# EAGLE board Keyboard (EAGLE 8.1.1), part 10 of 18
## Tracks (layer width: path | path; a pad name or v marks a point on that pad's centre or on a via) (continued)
S$9915 (continued)
  Bottom 0: 313.55,29.82 313.69,30.11
S$9916
  Bottom 0: 313.69,30.11 313.74,30.43
S$9917
  Bottom 0: 313.74,30.43 313.69,30.74
S$9918
  Bottom 0: 313.69,30.74 313.55,31.03
S$9919
  Bottom 0: 313.55,31.03 313.33,31.27
S$9920
  Bottom 0: 313.33,31.27 313.05,31.43
S$9921
  Bottom 0: 313.05,31.43 312.74,31.5
S$9922
  Bottom 0: 312.74,31.5 312.42,31.48
S$9923
  Bottom 0: 312.42,31.48 312.12,31.36
S$9924
  Bottom 0: 312.12,31.36 311.87,31.16
S$9925
  Bottom 0: 311.87,31.16 311.69,30.89
S$9926
  Bottom 0: 311.69,30.89 311.59,30.59
S$9927
  Bottom 0: 311.59,30.59 311.59,30.26
S$9928
  Bottom 0: 311.59,30.26 311.69,29.96
S$9929
  Bottom 0: 311.69,29.96 311.87,29.7
S$9930
  Bottom 0: 311.87,29.7 312.12,29.49
S$9931
  Bottom 0: 312.12,29.49 312.42,29.38
S$9932
  Bottom 0: 312.42,29.38 312.74,29.36
S$9933
  Bottom 0: 312.74,33.86 313.05,33.93
S$9934
  Bottom 0: 313.05,33.93 313.33,34.08
S$9935
  Bottom 0: 313.33,34.08 313.55,34.32
S$9936
  Bottom 0: 313.55,34.32 313.69,34.61
S$9937
  Bottom 0: 313.69,34.61 313.74,34.93
S$9938
  Bottom 0: 313.74,34.93 313.69,35.24
S$9939
  Bottom 0: 313.69,35.24 313.55,35.53
S$9940
  Bottom 0: 313.55,35.53 313.33,35.77
S$9941
  Bottom 0: 313.33,35.77 313.05,35.93
S$9942
  Bottom 0: 313.05,35.93 312.74,36
S$9943
  Bottom 0: 312.74,36 312.42,35.98
S$9944
  Bottom 0: 312.42,35.98 312.12,35.86
S$9945
  Bottom 0: 312.12,35.86 311.87,35.66
S$9946
  Bottom 0: 311.87,35.66 311.69,35.4
S$9947
  Bottom 0: 311.69,35.4 311.59,35.09
S$9948
  Bottom 0: 311.59,35.09 311.59,34.77
S$9949
  Bottom 0: 311.59,34.77 311.69,34.46
S$9950
  Bottom 0: 311.69,34.46 311.87,34.2
S$9951
  Bottom 0: 311.87,34.2 312.12,33.99
S$9952
  Bottom 0: 312.12,33.99 312.42,33.88
S$9953
  Bottom 0: 312.42,33.88 312.74,33.86
S$9954
  Bottom 0: 306.57,33.94 306.83,34.08
S$9955
  Bottom 0: 306.83,34.08 307.05,34.32
S$9956
  Bottom 0: 307.05,34.32 307.14,34.52
S$9957
  Bottom 0: 307.14,34.52 306.57,34.52
S$9958
  Bottom 0: 306.57,34.52 306.57,33.94
S$9959
  Bottom 0: 305.75,33.94 305.75,34.52
S$9960
  Bottom 0: 305.75,34.52 305.17,34.52
S$9961
  Bottom 0: 305.17,34.52 305.19,34.46
S$9962
  Bottom 0: 305.19,34.46 305.37,34.2
S$9963
  Bottom 0: 305.37,34.2 305.62,33.99
S$9964
  Bottom 0: 305.62,33.99 305.75,33.94
S$9965
  Bottom 0: 306.57,35.34 307.14,35.34
S$9966
  Bottom 0: 307.14,35.34 307.05,35.53
S$9967
  Bottom 0: 307.05,35.53 306.83,35.77
S$9968
  Bottom 0: 306.83,35.77 306.57,35.92
S$9969
  Bottom 0: 306.57,35.92 306.57,35.34
S$9970
  Bottom 0: 305.17,35.34 305.75,35.34
S$9971
  Bottom 0: 305.75,35.34 305.75,35.91
S$9972
  Bottom 0: 305.75,35.91 305.62,35.86
S$9973
  Bottom 0: 305.62,35.86 305.37,35.66
S$9974
  Bottom 0: 305.37,35.66 305.19,35.4
S$9975
  Bottom 0: 305.19,35.4 305.17,35.34
S$9976
  Bottom 0: 301.75,36.84 302.07,36.86
S$9977
  Bottom 0: 302.07,36.86 302.38,36.97
S$9978
  Bottom 0: 302.38,36.97 302.64,37.16
S$9979
  Bottom 0: 302.64,37.16 302.85,37.41
S$9980
  Bottom 0: 302.85,37.41 302.98,37.71
S$9981
  Bottom 0: 302.98,37.71 303.02,38.03
S$9982
  Bottom 0: 303.02,38.03 302.98,38.35
S$9983
  Bottom 0: 302.98,38.35 302.85,38.65
S$9984
  Bottom 0: 302.85,38.65 302.64,38.91
S$9985
  Bottom 0: 302.64,38.91 302.38,39.09
S$9986
  Bottom 0: 302.38,39.09 302.07,39.2
S$9987
  Bottom 0: 302.07,39.2 301.75,39.22
S$9988
  Bottom 0: 301.75,39.22 301.43,39.15
S$9989
  Bottom 0: 301.43,39.15 301.14,39.01
S$9990
  Bottom 0: 301.14,39.01 300.91,38.78
S$9991
  Bottom 0: 300.91,38.78 300.73,38.51
S$9992
  Bottom 0: 300.73,38.51 300.65,38.19
S$9993
  Bottom 0: 300.65,38.19 300.65,37.87
S$9994
  Bottom 0: 300.65,37.87 300.73,37.55
S$9995
  Bottom 0: 300.73,37.55 300.91,37.28
S$9996
  Bottom 0: 300.91,37.28 301.14,37.06
S$9997
  Bottom 0: 301.14,37.06 301.43,36.91
S$9998
  Bottom 0: 301.43,36.91 301.75,36.84
S$9999
  Bottom 0: 304.29,36.84 304.62,36.86
S$10000
  Bottom 0: 304.62,36.86 304.92,36.97
S$10001
  Bottom 0: 304.92,36.97 305.18,37.16
S$10002
  Bottom 0: 305.18,37.16 305.39,37.41
S$10003
  Bottom 0: 305.39,37.41 305.52,37.71
S$10004
  Bottom 0: 305.52,37.71 305.56,38.03
S$10005
  Bottom 0: 305.56,38.03 305.52,38.35
S$10006
  Bottom 0: 305.52,38.35 305.39,38.65
S$10007
  Bottom 0: 305.39,38.65 305.18,38.91
S$10008
  Bottom 0: 305.18,38.91 304.92,39.09
S$10009
  Bottom 0: 304.92,39.09 304.62,39.2
S$10010
  Bottom 0: 304.62,39.2 304.29,39.22
S$10011
  Bottom 0: 304.29,39.22 303.97,39.15
S$10012
  Bottom 0: 303.97,39.15 303.68,39.01
S$10013
  Bottom 0: 303.68,39.01 303.45,38.78
S$10014
  Bottom 0: 303.45,38.78 303.27,38.51
S$10015
  Bottom 0: 303.27,38.51 303.19,38.19
S$10016
  Bottom 0: 303.19,38.19 303.19,37.87
S$10017
  Bottom 0: 303.19,37.87 303.27,37.55
S$10018
  Bottom 0: 303.27,37.55 303.45,37.28
S$10019
  Bottom 0: 303.45,37.28 303.68,37.06
S$10020
  Bottom 0: 303.68,37.06 303.97,36.91
S$10021
  Bottom 0: 303.97,36.91 304.29,36.84
S$10022
  Bottom 0: 309.37,36.84 309.69,36.86
S$10023
  Bottom 0: 309.69,36.86 310,36.97
S$10024
  Bottom 0: 310,36.97 310.26,37.16
S$10025
  Bottom 0: 310.26,37.16 310.47,37.41
S$10026
  Bottom 0: 310.47,37.41 310.6,37.71
S$10027
  Bottom 0: 310.6,37.71 310.64,38.03
S$10028
  Bottom 0: 310.64,38.03 310.6,38.35
S$10029
  Bottom 0: 310.6,38.35 310.47,38.65
S$10030
  Bottom 0: 310.47,38.65 310.26,38.91
S$10031
  Bottom 0: 310.26,38.91 310,39.09
S$10032
  Bottom 0: 310,39.09 309.69,39.2
S$10033
  Bottom 0: 309.69,39.2 309.37,39.22
S$10034
  Bottom 0: 309.37,39.22 309.05,39.15
S$10035
  Bottom 0: 309.05,39.15 308.76,39.01
S$10036
  Bottom 0: 308.76,39.01 308.53,38.78
S$10037
  Bottom 0: 308.53,38.78 308.35,38.51
S$10038
  Bottom 0: 308.35,38.51 308.27,38.19
S$10039
  Bottom 0: 308.27,38.19 308.27,37.87
S$10040
  Bottom 0: 308.27,37.87 308.35,37.55
S$10041
  Bottom 0: 308.35,37.55 308.53,37.28
S$10042
  Bottom 0: 308.53,37.28 308.76,37.06
S$10043
  Bottom 0: 308.76,37.06 309.05,36.91
S$10044
  Bottom 0: 309.05,36.91 309.37,36.84
S$10045
  Bottom 0: 289.6,36.94 289.68,36.97
S$10046
  Bottom 0: 289.68,36.97 289.94,37.16
S$10047
  Bottom 0: 289.94,37.16 290.15,37.41
S$10048
  Bottom 0: 290.15,37.41 290.21,37.56
S$10049
  Bottom 0: 290.21,37.56 289.6,37.56
S$10050
  Bottom 0: 289.6,37.56 289.6,36.94
S$10051
  Bottom 0: 288.66,36.94 288.66,37.56
S$10052
  Bottom 0: 288.66,37.56 288.03,37.56
S$10053
  Bottom 0: 288.03,37.56 288.03,37.55
S$10054
  Bottom 0: 288.03,37.55 288.21,37.28
S$10055
  Bottom 0: 288.21,37.28 288.44,37.06
S$10056
  Bottom 0: 288.44,37.06 288.66,36.94
S$10057
  Bottom 0: 289.6,38.5 290.21,38.5
S$10058
  Bottom 0: 290.21,38.5 290.15,38.65
S$10059
  Bottom 0: 290.15,38.65 289.94,38.91
S$10060
  Bottom 0: 289.94,38.91 289.68,39.09
S$10061
  Bottom 0: 289.68,39.09 289.6,39.12
S$10062
  Bottom 0: 289.6,39.12 289.6,38.5
S$10063
  Bottom 0: 288.03,38.5 288.66,38.5
S$10064
  Bottom 0: 288.66,38.5 288.66,39.12
S$10065
  Bottom 0: 288.66,39.12 288.44,39.01
S$10066
  Bottom 0: 288.44,39.01 288.21,38.78
S$10067
  Bottom 0: 288.21,38.78 288.03,38.51
S$10068
  Bottom 0: 288.03,38.51 288.03,38.5
S$10069
  Bottom 0: 292.8,40.93 293.05,40.99
S$10070
  Bottom 0: 293.05,40.99 293.25,41.15
S$10071
  Bottom 0: 293.25,41.15 293.38,41.36
S$10072
  Bottom 0: 293.38,41.36 293.43,41.6
S$10073
  Bottom 0: 293.43,41.6 293.38,41.86
S$10074
  Bottom 0: 293.38,41.86 293.25,42.07
S$10075
  Bottom 0: 293.25,42.07 293.18,42.12
S$10076
  Bottom 0: 293.18,42.12 293.18,43.99
S$10077
  Bottom 0: 293.18,43.99 301.37,52.18
S$10078
  Bottom 0: 301.37,52.18 301.43,52.15
S$10079
  Bottom 0: 301.43,52.15 301.75,52.08
S$10080
  Bottom 0: 301.75,52.08 302.07,52.1
S$10081
  Bottom 0: 302.07,52.1 302.38,52.21
S$10082
  Bottom 0: 302.38,52.21 302.64,52.4
S$10083
  Bottom 0: 302.64,52.4 302.85,52.65
S$10084
  Bottom 0: 302.85,52.65 302.98,52.95
S$10085
  Bottom 0: 302.98,52.95 303.02,53.27
S$10086
  Bottom 0: 303.02,53.27 302.98,53.59
S$10087
  Bottom 0: 302.98,53.59 302.85,53.89
S$10088
  Bottom 0: 302.85,53.89 302.64,54.15
S$10089
  Bottom 0: 302.64,54.15 302.38,54.33
S$10090
  Bottom 0: 302.38,54.33 302.07,54.44
S$10091
  Bottom 0: 302.07,54.44 301.75,54.46
S$10092
  Bottom 0: 301.75,54.46 301.43,54.39
S$10093
  Bottom 0: 301.43,54.39 301.14,54.24
S$10094
  Bottom 0: 301.14,54.24 300.91,54.02
S$10095
  Bottom 0: 300.91,54.02 300.73,53.75
S$10096
  Bottom 0: 300.73,53.75 300.65,53.43
S$10097
  Bottom 0: 300.65,53.43 300.65,53.11
S$10098
  Bottom 0: 300.65,53.11 300.73,52.8
S$10099
  Bottom 0: 300.73,52.8 292.42,44.5
S$10100
  Bottom 0: 292.42,44.5 292.34,44.39
S$10101
  Bottom 0: 292.34,44.39 292.31,44.32
S$10102
  Bottom 0: 292.31,44.32 292.3,44.25
S$10103
  Bottom 0: 292.3,44.25 292.3,44.18
S$10104
  Bottom 0: 292.3,44.18 292.3,42.11
S$10105
  Bottom 0: 292.3,42.11 292.16,41.97
S$10106
  Bottom 0: 292.16,41.97 292.06,41.73
S$10107
  Bottom 0: 292.06,41.73 292.06,41.48
S$10108
  Bottom 0: 292.06,41.48 292.16,41.25
S$10109
  Bottom 0: 292.16,41.25 292.33,41.06
S$10110
  Bottom 0: 292.33,41.06 292.56,40.95
S$10111
  Bottom 0: 292.56,40.95 292.8,40.93
S$10112
  Bottom 0: 311.91,52.08 312.24,52.1
S$10113
  Bottom 0: 312.24,52.1 312.54,52.21
S$10114
  Bottom 0: 312.54,52.21 312.8,52.4
S$10115
  Bottom 0: 312.8,52.4 313.01,52.65
S$10116
  Bottom 0: 313.01,52.65 313.14,52.95
S$10117
  Bottom 0: 313.14,52.95 313.19,53.27
S$10118
  Bottom 0: 313.19,53.27 313.14,53.59
S$10119
  Bottom 0: 313.14,53.59 313.01,53.89
S$10120
  Bottom 0: 313.01,53.89 312.8,54.15
S$10121
  Bottom 0: 312.8,54.15 312.54,54.33
S$10122
  Bottom 0: 312.54,54.33 312.24,54.44
S$10123
  Bottom 0: 312.24,54.44 311.91,54.46
S$10124
  Bottom 0: 311.91,54.46 311.59,54.39
S$10125
  Bottom 0: 311.59,54.39 311.3,54.24
S$10126
  Bottom 0: 311.3,54.24 311.07,54.02
S$10127
  Bottom 0: 311.07,54.02 310.89,53.75
S$10128
  Bottom 0: 310.89,53.75 310.81,53.43
S$10129
  Bottom 0: 310.81,53.43 310.81,53.11
S$10130
  Bottom 0: 310.81,53.11 310.89,52.79
S$10131
  Bottom 0: 310.89,52.79 311.07,52.52
S$10132
  Bottom 0: 311.07,52.52 311.3,52.3
S$10133
  Bottom 0: 311.3,52.3 311.59,52.15
S$10134
  Bottom 0: 311.59,52.15 311.91,52.08
S$10135
  Bottom 0: 309.37,52.08 309.69,52.1
S$10136
  Bottom 0: 309.69,52.1 310,52.21
S$10137
  Bottom 0: 310,52.21 310.26,52.4
S$10138
  Bottom 0: 310.26,52.4 310.47,52.65
S$10139
  Bottom 0: 310.47,52.65 310.6,52.95
S$10140
  Bottom 0: 310.6,52.95 310.64,53.27
S$10141
  Bottom 0: 310.64,53.27 310.6,53.59
S$10142
  Bottom 0: 310.6,53.59 310.47,53.89
S$10143
  Bottom 0: 310.47,53.89 310.26,54.15
S$10144
  Bottom 0: 310.26,54.15 310,54.33
S$10145
  Bottom 0: 310,54.33 309.69,54.44
S$10146
  Bottom 0: 309.69,54.44 309.37,54.46
S$10147
  Bottom 0: 309.37,54.46 309.05,54.39
S$10148
  Bottom 0: 309.05,54.39 308.76,54.24
S$10149
  Bottom 0: 308.76,54.24 308.53,54.02
S$10150
  Bottom 0: 308.53,54.02 308.35,53.75
S$10151
  Bottom 0: 308.35,53.75 308.27,53.43
S$10152
  Bottom 0: 308.27,53.43 308.27,53.11
S$10153
  Bottom 0: 308.27,53.11 308.35,52.79
S$10154
  Bottom 0: 308.35,52.79 308.53,52.52
S$10155
  Bottom 0: 308.53,52.52 308.76,52.3
S$10156
  Bottom 0: 308.76,52.3 309.05,52.15
S$10157
  Bottom 0: 309.05,52.15 309.37,52.08
S$10158
  Bottom 0: 299.21,52.08 299.54,52.1
S$10159
  Bottom 0: 299.54,52.1 299.84,52.21
S$10160
  Bottom 0: 299.84,52.21 300.1,52.4
S$10161
  Bottom 0: 300.1,52.4 300.31,52.65
S$10162
  Bottom 0: 300.31,52.65 300.44,52.95
S$10163
  Bottom 0: 300.44,52.95 300.49,53.27
S$10164
  Bottom 0: 300.49,53.27 300.44,53.59
S$10165
  Bottom 0: 300.44,53.59 300.38,53.73
S$10166
  Bottom 0: 300.38,53.73 301.41,54.77
S$10167
  Bottom 0: 301.41,54.77 301.45,54.83
S$10168
  Bottom 0: 301.45,54.83 301.5,54.88
S$10169
  Bottom 0: 301.5,54.88 301.52,54.95
S$10170
  Bottom 0: 301.52,54.95 301.54,55.01
S$10171
  Bottom 0: 301.54,55.01 301.54,55.09
S$10172
  Bottom 0: 301.54,55.09 301.54,60.8
S$10173
  Bottom 0: 301.54,60.8 301.6,60.78
S$10174
  Bottom 0: 301.6,60.78 301.95,60.76
S$10175
  Bottom 0: 301.95,60.76 302.29,60.82
S$10176
  Bottom 0: 302.29,60.82 302.61,60.97
S$10177
  Bottom 0: 302.61,60.97 302.88,61.2
S$10178
  Bottom 0: 302.88,61.2 303.09,61.48
S$10179
  Bottom 0: 303.09,61.48 303.21,61.81
S$10180
  Bottom 0: 303.21,61.81 303.26,62.15
S$10181
  Bottom 0: 303.26,62.15 303.21,62.49
S$10182
  Bottom 0: 303.21,62.49 303.09,62.82
S$10183
  Bottom 0: 303.09,62.82 302.88,63.11
S$10184
  Bottom 0: 302.88,63.11 302.61,63.33
S$10185
  Bottom 0: 302.61,63.33 302.29,63.48
S$10186
  Bottom 0: 302.29,63.48 301.95,63.54
S$10187
  Bottom 0: 301.95,63.54 301.6,63.52
S$10188
  Bottom 0: 301.6,63.52 301.49,63.49
S$10189
  Bottom 0: 301.49,63.49 301.19,63.54
S$10190
  Bottom 0: 301.19,63.54 300.83,63.52
S$10191
  Bottom 0: 300.83,63.52 300.5,63.41
S$10192
  Bottom 0: 300.5,63.41 300.21,63.23
S$10193
  Bottom 0: 300.21,63.23 299.97,62.97
S$10194
  Bottom 0: 299.97,62.97 299.8,62.66
S$10195
  Bottom 0: 299.8,62.66 299.71,62.32
S$10196
  Bottom 0: 299.71,62.32 299.71,61.98
S$10197
  Bottom 0: 299.71,61.98 299.8,61.64
S$10198
  Bottom 0: 299.8,61.64 299.97,61.33
S$10199
  Bottom 0: 299.97,61.33 300.21,61.07
S$10200
  Bottom 0: 300.21,61.07 300.5,60.89
S$10201
  Bottom 0: 300.5,60.89 300.66,60.84
S$10202
  Bottom 0: 300.66,60.84 300.66,55.27
S$10203
  Bottom 0: 300.66,55.27 299.75,54.36
S$10204
  Bottom 0: 299.75,54.36 299.54,54.44
S$10205
  Bottom 0: 299.54,54.44 299.21,54.46
S$10206
  Bottom 0: 299.21,54.46 298.89,54.39
S$10207
  Bottom 0: 298.89,54.39 298.6,54.24
S$10208
  Bottom 0: 298.6,54.24 298.37,54.02
S$10209
  Bottom 0: 298.37,54.02 298.19,53.75
S$10210
  Bottom 0: 298.19,53.75 298.11,53.43
S$10211
  Bottom 0: 298.11,53.43 298.11,53.11
S$10212
  Bottom 0: 298.11,53.11 298.19,52.79
S$10213
  Bottom 0: 298.19,52.79 298.37,52.52
S$10214
  Bottom 0: 298.37,52.52 298.6,52.3
S$10215
  Bottom 0: 298.6,52.3 298.89,52.15
S$10216
  Bottom 0: 298.89,52.15 299.21,52.08
S$10217
  Bottom 0: 296.67,52.08 297,52.1
S$10218
  Bottom 0: 297,52.1 297.3,52.21
S$10219
  Bottom 0: 297.3,52.21 297.56,52.4
S$10220
  Bottom 0: 297.56,52.4 297.77,52.65
S$10221
  Bottom 0: 297.77,52.65 297.9,52.95
S$10222
  Bottom 0: 297.9,52.95 297.94,53.27
S$10223
  Bottom 0: 297.94,53.27 297.9,53.59
S$10224
  Bottom 0: 297.9,53.59 297.77,53.89
S$10225
  Bottom 0: 297.77,53.89 297.56,54.15
S$10226
  Bottom 0: 297.56,54.15 297.3,54.33
S$10227
  Bottom 0: 297.3,54.33 297,54.44
S$10228
  Bottom 0: 297,54.44 296.67,54.46
S$10229
  Bottom 0: 296.67,54.46 296.35,54.39
S$10230
  Bottom 0: 296.35,54.39 296.06,54.24
S$10231
  Bottom 0: 296.06,54.24 295.83,54.02
S$10232
  Bottom 0: 295.83,54.02 295.65,53.75
S$10233
  Bottom 0: 295.65,53.75 295.57,53.43
S$10234
  Bottom 0: 295.57,53.43 295.57,53.11
S$10235
  Bottom 0: 295.57,53.11 295.65,52.79
S$10236
  Bottom 0: 295.65,52.79 295.83,52.52
S$10237
  Bottom 0: 295.83,52.52 296.06,52.3
S$10238
  Bottom 0: 296.06,52.3 296.35,52.15
S$10239
  Bottom 0: 296.35,52.15 296.67,52.08
S$10240
  Bottom 0: 289.05,52.08 289.38,52.1
S$10241
  Bottom 0: 289.38,52.1 289.68,52.21
S$10242
  Bottom 0: 289.68,52.21 289.94,52.4
S$10243
  Bottom 0: 289.94,52.4 290.15,52.65
S$10244
  Bottom 0: 290.15,52.65 290.28,52.95
S$10245
  Bottom 0: 290.28,52.95 290.32,53.27
S$10246
  Bottom 0: 290.32,53.27 290.28,53.59
S$10247
  Bottom 0: 290.28,53.59 290.15,53.89
S$10248
  Bottom 0: 290.15,53.89 289.94,54.15
S$10249
  Bottom 0: 289.94,54.15 289.68,54.33
S$10250
  Bottom 0: 289.68,54.33 289.38,54.44
S$10251
  Bottom 0: 289.38,54.44 289.05,54.46
S$10252
  Bottom 0: 289.05,54.46 288.73,54.39
S$10253
  Bottom 0: 288.73,54.39 288.44,54.24
S$10254
  Bottom 0: 288.44,54.24 288.21,54.02
S$10255
  Bottom 0: 288.21,54.02 288.03,53.75
S$10256
  Bottom 0: 288.03,53.75 287.95,53.43
S$10257
  Bottom 0: 287.95,53.43 287.95,53.11
S$10258
  Bottom 0: 287.95,53.11 288.03,52.79
S$10259
  Bottom 0: 288.03,52.79 288.21,52.52
S$10260
  Bottom 0: 288.21,52.52 288.44,52.3
S$10261
  Bottom 0: 288.44,52.3 288.73,52.15
S$10262
  Bottom 0: 288.73,52.15 289.05,52.08
S$10263
  Bottom 0: 286.51,52.08 286.83,52.1
S$10264
  Bottom 0: 286.83,52.1 287.14,52.21
S$10265
  Bottom 0: 287.14,52.21 287.4,52.4
S$10266
  Bottom 0: 287.4,52.4 287.61,52.65
S$10267
  Bottom 0: 287.61,52.65 287.74,52.95
S$10268
  Bottom 0: 287.74,52.95 287.79,53.27
S$10269
  Bottom 0: 287.79,53.27 287.74,53.59
S$10270
  Bottom 0: 287.74,53.59 287.61,53.89
S$10271
  Bottom 0: 287.61,53.89 287.4,54.15
S$10272
  Bottom 0: 287.4,54.15 287.14,54.33
S$10273
  Bottom 0: 287.14,54.33 286.83,54.44
S$10274
  Bottom 0: 286.83,54.44 286.51,54.46
S$10275
  Bottom 0: 286.51,54.46 286.19,54.39
S$10276
  Bottom 0: 286.19,54.39 285.9,54.24
S$10277
  Bottom 0: 285.9,54.24 285.67,54.02
S$10278
  Bottom 0: 285.67,54.02 285.49,53.75
S$10279
  Bottom 0: 285.49,53.75 285.41,53.43
S$10280
  Bottom 0: 285.41,53.43 285.41,53.11
S$10281
  Bottom 0: 285.41,53.11 285.49,52.79
S$10282
  Bottom 0: 285.49,52.79 285.67,52.52
S$10283
  Bottom 0: 285.67,52.52 285.9,52.3
S$10284
  Bottom 0: 285.9,52.3 286.19,52.15
S$10285
  Bottom 0: 286.19,52.15 286.51,52.08
S$10286
  Bottom 0: 294.68,52.18 294.76,52.21
S$10287
  Bottom 0: 294.76,52.21 295.02,52.4
S$10288
  Bottom 0: 295.02,52.4 295.23,52.65
S$10289
  Bottom 0: 295.23,52.65 295.3,52.8
S$10290
  Bottom 0: 295.3,52.8 294.68,52.8
S$10291
  Bottom 0: 294.68,52.8 294.68,52.18
S$10292
  Bottom 0: 292.14,52.18 292.22,52.21
S$10293
  Bottom 0: 292.22,52.21 292.48,52.4
S$10294
  Bottom 0: 292.48,52.4 292.69,52.65
S$10295
  Bottom 0: 292.69,52.65 292.75,52.8
S$10296
  Bottom 0: 292.75,52.8 292.14,52.8
S$10297
  Bottom 0: 292.14,52.8 292.14,52.18
S$10298
  Bottom 0: 293.74,52.18 293.74,52.8
S$10299
  Bottom 0: 293.74,52.8 293.11,52.8
S$10300
  Bottom 0: 293.11,52.8 293.11,52.79
S$10301
  Bottom 0: 293.11,52.79 293.29,52.52
S$10302
  Bottom 0: 293.29,52.52 293.52,52.3
S$10303
  Bottom 0: 293.52,52.3 293.74,52.18
S$10304
  Bottom 0: 291.2,52.18 291.2,52.8
S$10305
  Bottom 0: 291.2,52.8 290.57,52.8
S$10306
  Bottom 0: 290.57,52.8 290.57,52.79
S$10307
  Bottom 0: 290.57,52.79 290.75,52.52
S$10308
  Bottom 0: 290.75,52.52 290.98,52.3
S$10309
  Bottom 0: 290.98,52.3 291.2,52.18
S$10310
  Bottom 0: 294.68,53.74 295.3,53.74
S$10311
  Bottom 0: 295.3,53.74 295.23,53.89
S$10312
  Bottom 0: 295.23,53.89 295.02,54.15
S$10313
  Bottom 0: 295.02,54.15 294.76,54.33
S$10314
  Bottom 0: 294.76,54.33 294.68,54.36
S$10315
  Bottom 0: 294.68,54.36 294.68,53.74
S$10316
  Bottom 0: 293.11,53.74 293.74,53.74
S$10317
  Bottom 0: 293.74,53.74 293.74,54.36
S$10318
  Bottom 0: 293.74,54.36 293.52,54.24
S$10319
  Bottom 0: 293.52,54.24 293.29,54.02
S$10320
  Bottom 0: 293.29,54.02 293.11,53.75
S$10321
  Bottom 0: 293.11,53.75 293.11,53.74
S$10322
  Bottom 0: 292.14,53.74 292.75,53.74
S$10323
  Bottom 0: 292.75,53.74 292.69,53.89
S$10324
  Bottom 0: 292.69,53.89 292.48,54.15
S$10325
  Bottom 0: 292.48,54.15 292.22,54.33
S$10326
  Bottom 0: 292.22,54.33 292.14,54.36
S$10327
  Bottom 0: 292.14,54.36 292.14,53.74
S$10328
  Bottom 0: 290.57,53.74 291.2,53.74
S$10329
  Bottom 0: 291.2,53.74 291.2,54.36
S$10330
  Bottom 0: 291.2,54.36 290.98,54.24
S$10331
  Bottom 0: 290.98,54.24 290.75,54.02
S$10332
  Bottom 0: 290.75,54.02 290.57,53.75
S$10333
  Bottom 0: 290.57,53.75 290.57,53.74
S$10334
  Bottom 0: 294.84,58.22 295.14,58.27
S$10335
  Bottom 0: 295.14,58.27 295.25,58.24
S$10336
  Bottom 0: 295.25,58.24 295.6,58.22
S$10337
  Bottom 0: 295.6,58.22 295.94,58.28
S$10338
  Bottom 0: 295.94,58.28 296.25,58.43
S$10339
  Bottom 0: 296.25,58.43 296.53,58.66
S$10340
  Bottom 0: 296.53,58.66 296.74,58.94
S$10341
  Bottom 0: 296.74,58.94 296.86,59.27
S$10342
  Bottom 0: 296.86,59.27 296.91,59.61
S$10343
  Bottom 0: 296.91,59.61 296.86,59.95
S$10344
  Bottom 0: 296.86,59.95 296.74,60.28
S$10345
  Bottom 0: 296.74,60.28 296.53,60.57
S$10346
  Bottom 0: 296.53,60.57 296.25,60.79
S$10347
  Bottom 0: 296.25,60.79 295.94,60.94
S$10348
  Bottom 0: 295.94,60.94 295.6,61
S$10349
  Bottom 0: 295.6,61 295.25,60.98
S$10350
  Bottom 0: 295.25,60.98 295.14,60.95
S$10351
  Bottom 0: 295.14,60.95 294.84,61
S$10352
  Bottom 0: 294.84,61 294.49,60.98
S$10353
  Bottom 0: 294.49,60.98 294.15,60.87
S$10354
  Bottom 0: 294.15,60.87 293.86,60.69
S$10355
  Bottom 0: 293.86,60.69 293.62,60.43
S$10356
  Bottom 0: 293.62,60.43 293.45,60.12
S$10357
  Bottom 0: 293.45,60.12 293.43,60.05
S$10358
  Bottom 0: 293.43,60.05 290.28,60.05
S$10359
  Bottom 0: 290.28,60.05 289.52,60.8
S$10360
  Bottom 0: 289.52,60.8 289.54,60.83
S$10361
  Bottom 0: 289.54,60.83 289.58,61.13
S$10362
  Bottom 0: 289.58,61.13 289.54,61.43
S$10363
  Bottom 0: 289.54,61.43 289.41,61.7
S$10364
  Bottom 0: 289.41,61.7 289.2,61.92
S$10365
  Bottom 0: 289.2,61.92 288.94,62.08
S$10366
  Bottom 0: 288.94,62.08 288.65,62.14
S$10367
  Bottom 0: 288.65,62.14 288.34,62.12
S$10368
  Bottom 0: 288.34,62.12 288.06,62.01
S$10369
  Bottom 0: 288.06,62.01 287.82,61.82
S$10370
  Bottom 0: 287.82,61.82 287.66,61.57
S$10371
  Bottom 0: 287.66,61.57 287.57,61.28
S$10372
  Bottom 0: 287.57,61.28 287.57,60.98
S$10373
  Bottom 0: 287.57,60.98 287.66,60.69
S$10374
  Bottom 0: 287.66,60.69 287.82,60.44
S$10375
  Bottom 0: 287.82,60.44 288.06,60.25
S$10376
  Bottom 0: 288.06,60.25 288.34,60.14
S$10377
  Bottom 0: 288.34,60.14 288.65,60.12
S$10378
  Bottom 0: 288.65,60.12 288.9,60.17
S$10379
  Bottom 0: 288.9,60.17 289.77,59.3
S$10380
  Bottom 0: 289.77,59.3 289.83,59.26
S$10381
  Bottom 0: 289.83,59.26 289.89,59.22
S$10382
  Bottom 0: 289.89,59.22 289.95,59.19
S$10383
  Bottom 0: 289.95,59.19 290.02,59.17
S$10384
  Bottom 0: 290.02,59.17 290.09,59.17
S$10385
  Bottom 0: 290.09,59.17 293.43,59.17
S$10386
  Bottom 0: 293.43,59.17 293.45,59.1
S$10387
  Bottom 0: 293.45,59.1 293.62,58.79
S$10388
  Bottom 0: 293.62,58.79 293.86,58.53
S$10389
  Bottom 0: 293.86,58.53 294.15,58.35
S$10390
  Bottom 0: 294.15,58.35 294.49,58.24
S$10391
  Bottom 0: 294.49,58.24 294.84,58.22
S$10392
  Bottom 0: 297.29,62.41 297.67,62.45
S$10393
  Bottom 0: 297.67,62.45 298.05,62.41
S$10394
  Bottom 0: 298.05,62.41 298.5,62.45
S$10395
  Bottom 0: 298.5,62.45 298.92,62.58
S$10396
  Bottom 0: 298.92,62.58 299.32,62.79
S$10397
  Bottom 0: 299.32,62.79 299.67,63.08
S$10398
  Bottom 0: 299.67,63.08 299.95,63.42
S$10399
  Bottom 0: 299.95,63.42 300.16,63.82
S$10400
  Bottom 0: 300.16,63.82 300.29,64.24
S$10401
  Bottom 0: 300.29,64.24 300.34,64.69
S$10402
  Bottom 0: 300.34,64.69 300.29,65.14
S$10403
  Bottom 0: 300.29,65.14 300.16,65.56
S$10404
  Bottom 0: 300.16,65.56 299.95,65.96
S$10405
  Bottom 0: 299.95,65.96 299.67,66.3
S$10406
  Bottom 0: 299.67,66.3 299.32,66.59
S$10407
  Bottom 0: 299.32,66.59 298.92,66.81
S$10408
  Bottom 0: 298.92,66.81 298.5,66.93
S$10409
  Bottom 0: 298.5,66.93 298.05,66.98
S$10410
  Bottom 0: 298.05,66.98 297.67,66.94
S$10411
  Bottom 0: 297.67,66.94 297.29,66.98
S$10412
  Bottom 0: 297.29,66.98 296.84,66.93
S$10413
  Bottom 0: 296.84,66.93 296.42,66.81
S$10414
  Bottom 0: 296.42,66.81 296.02,66.59
S$10415
  Bottom 0: 296.02,66.59 295.67,66.3
S$10416
  Bottom 0: 295.67,66.3 295.39,65.96
S$10417
  Bottom 0: 295.39,65.96 295.17,65.56
S$10418
  Bottom 0: 295.17,65.56 295.05,65.14
S$10419
  Bottom 0: 295.05,65.14 295,64.69
S$10420
  Bottom 0: 295,64.69 295.05,64.24
S$10421
  Bottom 0: 295.05,64.24 295.17,63.82
S$10422
  Bottom 0: 295.17,63.82 295.39,63.42
S$10423
  Bottom 0: 295.39,63.42 295.67,63.08
S$10424
  Bottom 0: 295.67,63.08 296.02,62.79
S$10425
  Bottom 0: 296.02,62.79 296.42,62.58
S$10426
  Bottom 0: 296.42,62.58 296.84,62.45
S$10427
  Bottom 0: 296.84,62.45 297.29,62.41
S$10428
  Bottom 0: 288.65,67.74 288.94,67.81
S$10429
  Bottom 0: 288.94,67.81 289.2,67.95
S$10430
  Bottom 0: 289.2,67.95 289.41,68.18
S$10431
  Bottom 0: 289.41,68.18 289.54,68.45
S$10432
  Bottom 0: 289.54,68.45 289.58,68.75
S$10433
  Bottom 0: 289.58,68.75 289.54,69.05
S$10434
  Bottom 0: 289.54,69.05 289.41,69.32
S$10435
  Bottom 0: 289.41,69.32 289.2,69.54
S$10436
  Bottom 0: 289.2,69.54 288.94,69.69
S$10437
  Bottom 0: 288.94,69.69 288.65,69.76
S$10438
  Bottom 0: 288.65,69.76 288.34,69.74
S$10439
  Bottom 0: 288.34,69.74 288.06,69.63
S$10440
  Bottom 0: 288.06,69.63 287.82,69.44
S$10441
  Bottom 0: 287.82,69.44 287.66,69.19
S$10442
  Bottom 0: 287.66,69.19 287.57,68.9
S$10443
  Bottom 0: 287.57,68.9 287.57,68.59
S$10444
  Bottom 0: 287.57,68.59 287.66,68.31
S$10445
  Bottom 0: 287.66,68.31 287.82,68.06
S$10446
  Bottom 0: 287.82,68.06 288.06,67.87
S$10447
  Bottom 0: 288.06,67.87 288.34,67.76
S$10448
  Bottom 0: 288.34,67.76 288.65,67.74
S$10449
  Bottom 0: 284.32,73.98 284.86,73.98
S$10450
  Bottom 0: 284.86,73.98 284.94,73.99
S$10451
  Bottom 0: 284.94,73.99 285.01,74.03
S$10452
  Bottom 0: 285.01,74.03 285.06,74.08
S$10453
  Bottom 0: 285.06,74.08 285.1,74.16
S$10454
  Bottom 0: 285.1,74.16 285.11,74.23
S$10455
  Bottom 0: 285.11,74.23 285.11,74.53
S$10456
  Bottom 0: 285.11,74.53 284.32,74.53
S$10457
  Bottom 0: 284.32,74.53 284.32,73.98
S$10458
  Bottom 0: 282.7,73.98 283.24,73.98
S$10459
  Bottom 0: 283.24,73.98 283.24,74.53
S$10460
  Bottom 0: 283.24,74.53 282.44,74.53
S$10461
  Bottom 0: 282.44,74.53 282.44,74.23
S$10462
  Bottom 0: 282.44,74.23 282.46,74.16
S$10463
  Bottom 0: 282.46,74.16 282.5,74.08
S$10464
  Bottom 0: 282.5,74.08 282.55,74.03
S$10465
  Bottom 0: 282.55,74.03 282.62,73.99
S$10466
  Bottom 0: 282.62,73.99 282.7,73.98
S$10467
  Bottom 0: 284.32,75.13 285.11,75.13
S$10468
  Bottom 0: 285.11,75.13 285.11,75.43
S$10469
  Bottom 0: 285.11,75.43 285.1,75.51
S$10470
  Bottom 0: 285.1,75.51 285.06,75.58
S$10471
  Bottom 0: 285.06,75.58 285.01,75.63
S$10472
  Bottom 0: 285.01,75.63 284.94,75.67
S$10473
  Bottom 0: 284.94,75.67 284.86,75.68
S$10474
  Bottom 0: 284.86,75.68 284.32,75.68
S$10475
  Bottom 0: 284.32,75.68 284.32,75.13
S$10476
  Bottom 0: 282.44,75.13 283.24,75.13
S$10477
  Bottom 0: 283.24,75.13 283.24,75.68
S$10478
  Bottom 0: 283.24,75.68 282.7,75.68
S$10479
  Bottom 0: 282.7,75.68 282.62,75.67
S$10480
  Bottom 0: 282.62,75.67 282.55,75.63
S$10481
  Bottom 0: 282.55,75.63 282.5,75.58
S$10482
  Bottom 0: 282.5,75.58 282.46,75.51
S$10483
  Bottom 0: 282.46,75.51 282.44,75.43
S$10484
  Bottom 0: 282.44,75.43 282.44,75.13
S$10485
  Bottom 0: 306.59,78.25 307.11,78.25
S$10486
  Bottom 0: 307.11,78.25 307.61,78.34
S$10487
  Bottom 0: 307.61,78.34 308.11,78.5
S$10488
  Bottom 0: 308.11,78.5 308.56,78.75
S$10489
  Bottom 0: 308.56,78.75 308.97,79.07
S$10490
  Bottom 0: 308.97,79.07 309.32,79.45
S$10491
  Bottom 0: 309.32,79.45 309.61,79.88
S$10492
  Bottom 0: 309.61,79.88 309.82,80.36
S$10493
  Bottom 0: 309.82,80.36 309.94,80.86
S$10494
  Bottom 0: 309.94,80.86 309.98,81.37
S$10495
  Bottom 0: 309.98,81.37 309.94,81.89
S$10496
  Bottom 0: 309.94,81.89 309.82,82.39
S$10497
  Bottom 0: 309.82,82.39 309.61,82.87
S$10498
  Bottom 0: 309.61,82.87 309.32,83.3
S$10499
  Bottom 0: 309.32,83.3 308.97,83.68
S$10500
  Bottom 0: 308.97,83.68 308.56,84
S$10501
  Bottom 0: 308.56,84 308.11,84.24
S$10502
  Bottom 0: 308.11,84.24 307.61,84.41
S$10503
  Bottom 0: 307.61,84.41 307.11,84.5
S$10504
  Bottom 0: 307.11,84.5 306.59,84.5
S$10505
  Bottom 0: 306.59,84.5 306.08,84.41
S$10506
  Bottom 0: 306.08,84.41 305.59,84.24
S$10507
  Bottom 0: 305.59,84.24 305.14,84
S$10508
  Bottom 0: 305.14,84 304.73,83.68
S$10509
  Bottom 0: 304.73,83.68 304.38,83.3
S$10510
  Bottom 0: 304.38,83.3 304.09,82.87
S$10511
  Bottom 0: 304.09,82.87 303.88,82.39
S$10512
  Bottom 0: 303.88,82.39 303.76,81.89
S$10513
  Bottom 0: 303.76,81.89 303.71,81.37
S$10514
  Bottom 0: 303.71,81.37 303.76,80.86
S$10515
  Bottom 0: 303.76,80.86 303.88,80.36
S$10516
  Bottom 0: 303.88,80.36 304.09,79.88
S$10517
  Bottom 0: 304.09,79.88 304.38,79.45
S$10518
  Bottom 0: 304.38,79.45 304.73,79.07
S$10519
  Bottom 0: 304.73,79.07 305.14,78.75
S$10520
  Bottom 0: 305.14,78.75 305.59,78.5
S$10521
  Bottom 0: 305.59,78.5 306.08,78.34
S$10522
  Bottom 0: 306.08,78.34 306.59,78.25
S$10523
  Bottom 0: 289.84,79.65 290.14,79.72
S$10524
  Bottom 0: 290.14,79.72 290.4,79.87
S$10525
  Bottom 0: 290.4,79.87 290.6,80.09
S$10526
  Bottom 0: 290.6,80.09 290.74,80.36
S$10527
  Bottom 0: 290.74,80.36 290.78,80.66
S$10528
  Bottom 0: 290.78,80.66 290.74,80.96
S$10529
  Bottom 0: 290.74,80.96 290.6,81.24
S$10530
  Bottom 0: 290.6,81.24 290.4,81.45
S$10531
  Bottom 0: 290.4,81.45 290.14,81.61
S$10532
  Bottom 0: 290.14,81.61 289.84,81.67
S$10533
  Bottom 0: 289.84,81.67 289.54,81.65
S$10534
  Bottom 0: 289.54,81.65 289.26,81.54
S$10535
  Bottom 0: 289.26,81.54 289.02,81.35
S$10536
  Bottom 0: 289.02,81.35 288.85,81.11
S$10537
  Bottom 0: 288.85,81.11 288.76,80.81
S$10538
  Bottom 0: 288.76,80.81 288.76,80.51
S$10539
  Bottom 0: 288.76,80.51 288.85,80.22
S$10540
  Bottom 0: 288.85,80.22 289.02,79.97
S$10541
  Bottom 0: 289.02,79.97 289.26,79.78
S$10542
  Bottom 0: 289.26,79.78 289.54,79.67
S$10543
  Bottom 0: 289.54,79.67 289.84,79.65
S$10544
  Bottom 0: 287.52,82.63 287.52,83.12
S$10545
  Bottom 0: 287.52,83.12 287.03,83.12
S$10546
  Bottom 0: 287.03,83.12 287.07,83.02
S$10547
  Bottom 0: 287.07,83.02 287.24,82.79
S$10548
  Bottom 0: 287.24,82.79 287.48,82.64
S$10549
  Bottom 0: 287.48,82.64 287.52,82.63
S$10550
  Bottom 0: 288.12,82.63 288.29,82.7
S$10551
  Bottom 0: 288.29,82.7 288.5,82.9
S$10552
  Bottom 0: 288.5,82.9 288.62,83.12
S$10553
  Bottom 0: 288.62,83.12 288.12,83.12
S$10554
  Bottom 0: 288.12,83.12 288.12,82.63
S$10555
  Bottom 0: 288.12,83.72 288.62,83.72
S$10556
  Bottom 0: 288.62,83.72 288.5,83.94
S$10557
  Bottom 0: 288.5,83.94 288.29,84.14
S$10558
  Bottom 0: 288.29,84.14 288.12,84.21
S$10559
  Bottom 0: 288.12,84.21 288.12,83.72
S$10560
  Bottom 0: 289.3,87.25 289.3,87.95
S$10561
  Bottom 0: 289.3,87.95 288.6,87.95
S$10562
  Bottom 0: 288.6,87.95 288.75,87.7
S$10563
  Bottom 0: 288.75,87.7 288.98,87.44
S$10564
  Bottom 0: 288.98,87.44 289.28,87.26
S$10565
  Bottom 0: 289.28,87.26 289.3,87.25
S$10566
  Bottom 0: 290.45,87.26 290.63,87.34
S$10567
  Bottom 0: 290.63,87.34 290.9,87.57
S$10568
  Bottom 0: 290.9,87.57 291.1,87.85
S$10569
  Bottom 0: 291.1,87.85 291.15,87.95
S$10570
  Bottom 0: 291.15,87.95 290.45,87.95
S$10571
  Bottom 0: 290.45,87.95 290.45,87.26
S$10572
  Bottom 0: 59.95,12.5 59.98,12.64
S$10573
  Bottom 0: 59.98,12.64 59.93,12.96
S$10574
  Bottom 0: 59.93,12.96 59.79,13.26
S$10575
  Bottom 0: 59.79,13.26 59.58,13.5
S$10576
  Bottom 0: 59.58,13.5 59.31,13.68
S$10577
  Bottom 0: 59.31,13.68 59,13.77
S$10578
  Bottom 0: 59,13.77 58.67,13.77
S$10579
  Bottom 0: 58.67,13.77 58.54,13.73
S$10580
  Bottom 0: 58.54,13.73 56.56,15.71
S$10581
  Bottom 0: 56.56,15.71 56.56,27.38
S$10582
  Bottom 0: 56.56,27.38 56.56,27.48
S$10583
  Bottom 0: 56.56,27.48 56.54,27.56
S$10584
  Bottom 0: 56.54,27.56 56.5,27.64
S$10585
  Bottom 0: 56.5,27.64 56.46,27.72
S$10586
  Bottom 0: 56.46,27.72 56.39,27.79
S$10587
  Bottom 0: 56.39,27.79 52.79,31.39
S$10588
  Bottom 0: 52.79,31.39 52.83,31.69
S$10589
  Bottom 0: 52.83,31.69 52.78,32.01
S$10590
  Bottom 0: 52.78,32.01 52.65,32.31
S$10591
  Bottom 0: 52.65,32.31 52.43,32.55
S$10592
  Bottom 0: 52.43,32.55 52.16,32.73
S$10593
  Bottom 0: 52.16,32.73 51.85,32.82
S$10594
  Bottom 0: 51.85,32.82 51.52,32.82
S$10595
  Bottom 0: 51.52,32.82 51.21,32.73
S$10596
  Bottom 0: 51.21,32.73 50.94,32.55
S$10597
  Bottom 0: 50.94,32.55 50.73,32.31
S$10598
  Bottom 0: 50.73,32.31 50.59,32.01
S$10599
  Bottom 0: 50.59,32.01 50.54,31.69
S$10600
  Bottom 0: 50.54,31.69 50.59,31.37
S$10601
  Bottom 0: 50.59,31.37 50.73,31.07
S$10602
  Bottom 0: 50.73,31.07 50.94,30.82
S$10603
  Bottom 0: 50.94,30.82 51.21,30.64
S$10604
  Bottom 0: 51.21,30.64 51.52,30.55
S$10605
  Bottom 0: 51.52,30.55 51.85,30.55
S$10606
  Bottom 0: 51.85,30.55 51.98,30.59
S$10607
  Bottom 0: 51.98,30.59 55.42,27.15
S$10608
  Bottom 0: 55.42,27.15 55.42,24.77
S$10609
  Bottom 0: 55.42,24.77 55.24,25.02
S$10610
  Bottom 0: 55.24,25.02 54.97,25.25
S$10611
  Bottom 0: 54.97,25.25 54.67,25.39
S$10612
  Bottom 0: 54.67,25.39 54.67,26.2
S$10613
  Bottom 0: 54.67,26.2 54.66,26.28
S$10614
  Bottom 0: 54.66,26.28 54.65,26.34
S$10615
  Bottom 0: 54.65,26.34 54.62,26.4
S$10616
  Bottom 0: 54.62,26.4 54.58,26.46
S$10617
  Bottom 0: 54.58,26.46 54.54,26.52
S$10618
  Bottom 0: 54.54,26.52 50.8,30.25
S$10619
  Bottom 0: 50.8,30.25 50.75,30.3
S$10620
  Bottom 0: 50.75,30.3 50.69,30.34
S$10621
  Bottom 0: 50.69,30.34 50.63,30.36
S$10622
  Bottom 0: 50.63,30.36 50.56,30.38
S$10623
  Bottom 0: 50.56,30.38 50.49,30.38
S$10624
  Bottom 0: 50.49,30.38 46.93,30.38
S$10625
  Bottom 0: 46.93,30.38 38.11,39.2
S$10626
  Bottom 0: 38.11,39.2 38.44,39.19
S$10627
  Bottom 0: 38.44,39.19 38.78,39.25
S$10628
  Bottom 0: 38.78,39.25 39.1,39.4
S$10629
  Bottom 0: 39.1,39.4 39.37,39.62
S$10630
  Bottom 0: 39.37,39.62 39.57,39.91
S$10631
  Bottom 0: 39.57,39.91 39.7,40.23
S$10632
  Bottom 0: 39.7,40.23 39.75,40.58
S$10633
  Bottom 0: 39.75,40.58 39.7,40.92
S$10634
  Bottom 0: 39.7,40.92 39.57,41.25
S$10635
  Bottom 0: 39.57,41.25 39.37,41.53
S$10636
  Bottom 0: 39.37,41.53 39.1,41.76
S$10637
  Bottom 0: 39.1,41.76 38.78,41.91
S$10638
  Bottom 0: 38.78,41.91 38.44,41.97
S$10639
  Bottom 0: 38.44,41.97 38.09,41.95
S$10640
  Bottom 0: 38.09,41.95 37.76,41.84
S$10641
  Bottom 0: 37.76,41.84 37.46,41.65
S$10642
  Bottom 0: 37.46,41.65 37.28,41.46
S$10643
  Bottom 0: 37.28,41.46 37.28,44.86
S$10644
  Bottom 0: 37.28,44.86 38.7,46.29
S$10645
  Bottom 0: 38.7,46.29 38.65,46.1
S$10646
  Bottom 0: 38.65,46.1 38.6,45.66
S$10647
  Bottom 0: 38.6,45.66 38.65,45.21
S$10648
  Bottom 0: 38.65,45.21 38.78,44.78
S$10649
  Bottom 0: 38.78,44.78 38.99,44.39
S$10650
  Bottom 0: 38.99,44.39 39.28,44.04
S$10651
  Bottom 0: 39.28,44.04 39.62,43.76
S$10652
  Bottom 0: 39.62,43.76 40.02,43.54
S$10653
  Bottom 0: 40.02,43.54 40.44,43.42
S$10654
  Bottom 0: 40.44,43.42 40.89,43.37
S$10655
  Bottom 0: 40.89,43.37 41.34,43.42
S$10656
  Bottom 0: 41.34,43.42 41.76,43.54
S$10657
  Bottom 0: 41.76,43.54 42.16,43.76
S$10658
  Bottom 0: 42.16,43.76 42.51,44.04
S$10659
  Bottom 0: 42.51,44.04 42.79,44.39
S$10660
  Bottom 0: 42.79,44.39 43,44.78
S$10661
  Bottom 0: 43,44.78 43.13,45.21
S$10662
  Bottom 0: 43.13,45.21 43.18,45.66
S$10663
  Bottom 0: 43.18,45.66 43.13,46.1
S$10664
  Bottom 0: 43.13,46.1 43,46.53
S$10665
  Bottom 0: 43,46.53 42.79,46.93
S$10666
  Bottom 0: 42.79,46.93 42.51,47.27
S$10667
  Bottom 0: 42.51,47.27 42.16,47.56
S$10668
  Bottom 0: 42.16,47.56 41.76,47.77
S$10669
  Bottom 0: 41.76,47.77 41.34,47.89
S$10670
  Bottom 0: 41.34,47.89 40.89,47.94
S$10671
  Bottom 0: 40.89,47.94 40.44,47.89
S$10672
  Bottom 0: 40.44,47.89 40.26,47.84
S$10673
  Bottom 0: 40.26,47.84 41.21,48.8
S$10674
  Bottom 0: 41.21,48.8 41.25,48.84
S$10675
  Bottom 0: 41.25,48.84 41.29,48.91
S$10676
  Bottom 0: 41.29,48.91 41.32,48.97
S$10677
  Bottom 0: 41.32,48.97 41.33,49.03
S$10678
  Bottom 0: 41.33,49.03 41.34,49.1
S$10679
  Bottom 0: 41.34,49.1 41.34,49.96
S$10680
  Bottom 0: 41.34,49.96 41.41,49.87
S$10681
  Bottom 0: 41.41,49.87 41.69,49.7
S$10682
  Bottom 0: 41.69,49.7 42,49.6
S$10683
  Bottom 0: 42,49.6 42.32,49.6
S$10684
  Bottom 0: 42.32,49.6 42.63,49.7
S$10685
  Bottom 0: 42.63,49.7 42.91,49.87
S$10686
  Bottom 0: 42.91,49.87 43.12,50.11
S$10687
  Bottom 0: 43.12,50.11 43.26,50.42
S$10688
  Bottom 0: 43.26,50.42 43.3,50.74
S$10689
  Bottom 0: 43.3,50.74 43.26,51.06
S$10690
  Bottom 0: 43.26,51.06 43.12,51.36
S$10691
  Bottom 0: 43.12,51.36 42.91,51.6
S$10692
  Bottom 0: 42.91,51.6 42.63,51.78
S$10693
  Bottom 0: 42.63,51.78 42.32,51.87
S$10694
  Bottom 0: 42.32,51.87 42,51.87
S$10695
  Bottom 0: 42,51.87 41.69,51.78
S$10696
  Bottom 0: 41.69,51.78 41.41,51.6
S$10697
  Bottom 0: 41.41,51.6 41.34,51.51
S$10698
  Bottom 0: 41.34,51.51 41.34,53.72
S$10699
  Bottom 0: 41.34,53.72 41.49,53.86
S$10700
  Bottom 0: 41.49,53.86 41.5,53.87
S$10701
  Bottom 0: 41.5,53.87 43.47,55.83
S$10702
  Bottom 0: 43.47,55.83 45.73,55.83
S$10703
  Bottom 0: 45.73,55.83 45.02,55.13
S$10704
  Bottom 0: 45.02,55.13 44.95,55.16
S$10705
  Bottom 0: 44.95,55.16 44.62,55.18
S$10706
  Bottom 0: 44.62,55.18 44.3,55.12
S$10707
  Bottom 0: 44.3,55.12 44.01,54.97
S$10708
  Bottom 0: 44.01,54.97 43.78,54.74
S$10709
  Bottom 0: 43.78,54.74 43.61,54.47
S$10710
  Bottom 0: 43.61,54.47 43.52,54.16
S$10711
  Bottom 0: 43.52,54.16 43.52,53.83
S$10712
  Bottom 0: 43.52,53.83 43.61,53.52
S$10713
  Bottom 0: 43.61,53.52 43.78,53.24
S$10714
  Bottom 0: 43.78,53.24 44.01,53.02
S$10715
  Bottom 0: 44.01,53.02 44.3,52.87
S$10716
  Bottom 0: 44.3,52.87 44.62,52.8
S$10717
  Bottom 0: 44.62,52.8 44.95,52.82
S$10718
  Bottom 0: 44.95,52.82 45.25,52.93
S$10719
  Bottom 0: 45.25,52.93 45.52,53.12
S$10720
  Bottom 0: 45.52,53.12 45.73,53.37
S$10721
  Bottom 0: 45.73,53.37 45.85,53.67
S$10722
  Bottom 0: 45.85,53.67 45.9,53.99
S$10723
  Bottom 0: 45.9,53.99 45.88,54.08
S$10724
  Bottom 0: 45.88,54.08 46.02,53.95
S$10725
  Bottom 0: 46.02,53.95 46.02,51.72
S$10726
  Bottom 0: 46.02,51.72 46.02,51.65
S$10727
  Bottom 0: 46.02,51.65 46.04,51.58
S$10728
  Bottom 0: 46.04,51.58 46.06,51.52
S$10729
  Bottom 0: 46.06,51.52 46.1,51.46
S$10730
  Bottom 0: 46.1,51.46 46.14,51.41
S$10731
  Bottom 0: 46.14,51.41 54.75,42.8
S$10732
  Bottom 0: 54.75,42.8 54.81,42.76
S$10733
  Bottom 0: 54.81,42.76 54.87,42.72
S$10734
  Bottom 0: 54.87,42.72 54.93,42.69
S$10735
  Bottom 0: 54.93,42.69 54.99,42.68
S$10736
  Bottom 0: 54.99,42.68 55.06,42.67
S$10737
  Bottom 0: 55.06,42.67 62.43,42.67
S$10738
  Bottom 0: 62.43,42.67 62.46,42.6
S$10739
  Bottom 0: 62.46,42.6 62.63,42.29
S$10740
  Bottom 0: 62.63,42.29 62.87,42.04
S$10741
  Bottom 0: 62.87,42.04 63.16,41.85
S$10742
  Bottom 0: 63.16,41.85 63.49,41.74
S$10743
  Bottom 0: 63.49,41.74 63.84,41.73
S$10744
  Bottom 0: 63.84,41.73 64.19,41.79
S$10745
  Bottom 0: 64.19,41.79 64.5,41.94
S$10746
  Bottom 0: 64.5,41.94 64.77,42.16
S$10747
  Bottom 0: 64.77,42.16 64.98,42.45
S$10748
  Bottom 0: 64.98,42.45 65.11,42.77
S$10749
  Bottom 0: 65.11,42.77 65.15,43.12
S$10750
  Bottom 0: 65.15,43.12 65.11,43.46
S$10751
  Bottom 0: 65.11,43.46 64.98,43.79
S$10752
  Bottom 0: 64.98,43.79 64.77,44.07
S$10753
  Bottom 0: 64.77,44.07 64.5,44.3
S$10754
  Bottom 0: 64.5,44.3 64.19,44.45
S$10755
  Bottom 0: 64.19,44.45 63.84,44.51
S$10756
  Bottom 0: 63.84,44.51 63.49,44.49
S$10757
  Bottom 0: 63.49,44.49 63.16,44.38
S$10758
  Bottom 0: 63.16,44.38 62.87,44.19
S$10759
  Bottom 0: 62.87,44.19 62.63,43.94
S$10760
  Bottom 0: 62.63,43.94 62.46,43.63
S$10761
  Bottom 0: 62.46,43.63 62.43,43.56
S$10762
  Bottom 0: 62.43,43.56 60.85,43.56
S$10763
  Bottom 0: 60.85,43.56 61.22,43.76
S$10764
  Bottom 0: 61.22,43.76 61.56,44.04
S$10765
  Bottom 0: 61.56,44.04 61.85,44.39
S$10766
  Bottom 0: 61.85,44.39 62.06,44.78
S$10767
  Bottom 0: 62.06,44.78 62.19,45.21
S$10768
  Bottom 0: 62.19,45.21 62.23,45.66
S$10769
  Bottom 0: 62.23,45.66 62.19,46.1
S$10770
  Bottom 0: 62.19,46.1 62.06,46.53
S$10771
  Bottom 0: 62.06,46.53 61.85,46.93
S$10772
  Bottom 0: 61.85,46.93 61.56,47.27
S$10773
  Bottom 0: 61.56,47.27 61.22,47.56
S$10774
  Bottom 0: 61.22,47.56 60.82,47.77
S$10775
  Bottom 0: 60.82,47.77 60.39,47.89
S$10776
  Bottom 0: 60.39,47.89 59.95,47.94
S$10777
  Bottom 0: 59.95,47.94 59.5,47.89
S$10778
  Bottom 0: 59.5,47.89 59.07,47.77
S$10779
  Bottom 0: 59.07,47.77 58.68,47.56
S$10780
  Bottom 0: 58.68,47.56 58.33,47.27
S$10781
  Bottom 0: 58.33,47.27 58.04,46.93
S$10782
  Bottom 0: 58.04,46.93 57.83,46.53
S$10783
  Bottom 0: 57.83,46.53 57.71,46.1
S$10784
  Bottom 0: 57.71,46.1 57.66,45.66
S$10785
  Bottom 0: 57.66,45.66 57.71,45.21
S$10786
  Bottom 0: 57.71,45.21 57.83,44.78
S$10787
  Bottom 0: 57.83,44.78 58.04,44.39
S$10788
  Bottom 0: 58.04,44.39 58.33,44.04
S$10789
  Bottom 0: 58.33,44.04 58.68,43.76
S$10790
  Bottom 0: 58.68,43.76 59.04,43.56
S$10791
  Bottom 0: 59.04,43.56 55.25,43.56
S$10792
  Bottom 0: 55.25,43.56 50.04,48.77
S$10793
  Bottom 0: 50.04,48.77 50.19,48.71
S$10794
  Bottom 0: 50.19,48.71 50.49,48.69
S$10795
  Bottom 0: 50.49,48.69 50.79,48.76
S$10796
  Bottom 0: 50.79,48.76 51.06,48.91
S$10797
  Bottom 0: 51.06,48.91 51.09,48.95
S$10798
  Bottom 0: 51.09,48.95 68.8,48.95
S$10799
  Bottom 0: 68.8,48.95 68.96,48.82
S$10800
  Bottom 0: 68.96,48.82 69.24,48.71
S$10801
  Bottom 0: 69.24,48.71 69.55,48.69
S$10802
  Bottom 0: 69.55,48.69 69.84,48.76
S$10803
  Bottom 0: 69.84,48.76 70.11,48.91
S$10804
  Bottom 0: 70.11,48.91 70.31,49.13
S$10805
  Bottom 0: 70.31,49.13 70.44,49.4
S$10806
  Bottom 0: 70.44,49.4 70.48,49.66
S$10807
  Bottom 0: 70.48,49.66 78.41,41.74
S$10808
  Bottom 0: 78.41,41.74 78.41,40.87
S$10809
  Bottom 0: 78.41,40.87 77.81,40.27
S$10810
  Bottom 0: 77.81,40.27 77.85,40.58
S$10811
  Bottom 0: 77.85,40.58 77.8,40.92
S$10812
  Bottom 0: 77.8,40.92 77.67,41.25
S$10813
  Bottom 0: 77.67,41.25 77.47,41.53
S$10814
  Bottom 0: 77.47,41.53 77.2,41.76
S$10815
  Bottom 0: 77.2,41.76 76.88,41.91
S$10816
  Bottom 0: 76.88,41.91 76.54,41.97
S$10817
  Bottom 0: 76.54,41.97 76.19,41.95
S$10818
  Bottom 0: 76.19,41.95 75.86,41.84
S$10819
  Bottom 0: 75.86,41.84 75.83,41.83
S$10820
  Bottom 0: 75.83,41.83 75.26,42.4
S$10821
  Bottom 0: 75.26,42.4 75.21,42.43
S$10822
  Bottom 0: 75.21,42.43 75.15,42.48
S$10823
  Bottom 0: 75.15,42.48 75.08,42.5
S$10824
  Bottom 0: 75.08,42.5 75.02,42.52
S$10825
  Bottom 0: 75.02,42.52 74.95,42.52
S$10826
  Bottom 0: 74.95,42.52 70.38,42.52
S$10827
  Bottom 0: 70.38,42.52 70.31,42.65
S$10828
  Bottom 0: 70.31,42.65 70.11,42.87
S$10829
  Bottom 0: 70.11,42.87 69.84,43.02
S$10830
  Bottom 0: 69.84,43.02 69.55,43.09
S$10831
  Bottom 0: 69.55,43.09 69.24,43.07
S$10832
  Bottom 0: 69.24,43.07 68.96,42.96
S$10833
  Bottom 0: 68.96,42.96 68.72,42.77
S$10834
  Bottom 0: 68.72,42.77 68.56,42.52
S$10835
  Bottom 0: 68.56,42.52 68.46,42.23
S$10836
  Bottom 0: 68.46,42.23 68.46,41.92
S$10837
  Bottom 0: 68.46,41.92 68.56,41.64
S$10838
  Bottom 0: 68.56,41.64 68.72,41.39
S$10839
  Bottom 0: 68.72,41.39 68.96,41.2
S$10840
  Bottom 0: 68.96,41.2 69.24,41.09
S$10841
  Bottom 0: 69.24,41.09 69.55,41.07
S$10842
  Bottom 0: 69.55,41.07 69.84,41.13
S$10843
  Bottom 0: 69.84,41.13 70.11,41.28
S$10844
  Bottom 0: 70.11,41.28 70.31,41.51
S$10845
  Bottom 0: 70.31,41.51 70.38,41.64
S$10846
  Bottom 0: 70.38,41.64 74.76,41.64
S$10847
  Bottom 0: 74.76,41.64 75.21,41.19
S$10848
  Bottom 0: 75.21,41.19 75.15,41.09
S$10849
  Bottom 0: 75.15,41.09 75.06,40.75
S$10850
  Bottom 0: 75.06,40.75 75.06,40.4
S$10851
  Bottom 0: 75.06,40.4 75.15,40.06
S$10852
  Bottom 0: 75.15,40.06 75.32,39.75
S$10853
  Bottom 0: 75.32,39.75 75.56,39.5
S$10854
  Bottom 0: 75.56,39.5 75.86,39.31
S$10855
  Bottom 0: 75.86,39.31 76.19,39.2
S$10856
  Bottom 0: 76.19,39.2 76.54,39.19
S$10857
  Bottom 0: 76.54,39.19 76.77,39.23
S$10858
  Bottom 0: 76.77,39.23 73.62,36.08
S$10859
  Bottom 0: 73.62,36.08 73.53,36.11
S$10860
  Bottom 0: 73.53,36.11 73.2,36.13
S$10861
  Bottom 0: 73.2,36.13 72.89,36.06
S$10862
  Bottom 0: 72.89,36.06 72.59,35.91
S$10863
  Bottom 0: 72.59,35.91 72.36,35.69
S$10864
  Bottom 0: 72.36,35.69 72.19,35.41
S$10865
  Bottom 0: 72.19,35.41 72.1,35.1
S$10866
  Bottom 0: 72.1,35.1 72.1,34.77
S$10867
  Bottom 0: 72.1,34.77 72.19,34.46
S$10868
  Bottom 0: 72.19,34.46 72.36,34.19
S$10869
  Bottom 0: 72.36,34.19 72.59,33.96
S$10870
  Bottom 0: 72.59,33.96 72.89,33.81
S$10871
  Bottom 0: 72.89,33.81 73.2,33.75
S$10872
  Bottom 0: 73.2,33.75 73.53,33.77
S$10873
  Bottom 0: 73.53,33.77 73.83,33.88
S$10874
  Bottom 0: 73.83,33.88 74.1,34.06
S$10875
  Bottom 0: 74.1,34.06 74.31,34.32
S$10876
  Bottom 0: 74.31,34.32 74.43,34.62
S$10877
  Bottom 0: 74.43,34.62 74.48,34.94
S$10878
  Bottom 0: 74.48,34.94 74.43,35.26
S$10879
  Bottom 0: 74.43,35.26 74.42,35.28
S$10880
  Bottom 0: 74.42,35.28 79.38,40.24
S$10881
  Bottom 0: 79.38,40.24 79.44,40.3
S$10882
  Bottom 0: 79.44,40.3 79.49,40.38
S$10883
  Bottom 0: 79.49,40.38 79.53,40.46
S$10884
  Bottom 0: 79.53,40.46 79.54,40.55
S$10885
  Bottom 0: 79.54,40.55 79.55,40.64
S$10886
  Bottom 0: 79.55,40.64 79.55,41.51
S$10887
  Bottom 0: 79.55,41.51 79.56,41.51
S$10888
  Bottom 0: 79.56,41.51 79.63,41.57
S$10889
  Bottom 0: 79.63,41.57 81.44,43.38
S$10890
  Bottom 0: 81.44,43.38 81.41,43.29
S$10891
  Bottom 0: 81.41,43.29 81.41,42.94
S$10892
  Bottom 0: 81.41,42.94 81.5,42.6
S$10893
  Bottom 0: 81.5,42.6 81.67,42.29
S$10894
  Bottom 0: 81.67,42.29 81.91,42.04
S$10895
  Bottom 0: 81.91,42.04 82.2,41.85
S$10896
  Bottom 0: 82.2,41.85 82.54,41.74
S$10897
  Bottom 0: 82.54,41.74 82.89,41.73
S$10898
  Bottom 0: 82.89,41.73 83.23,41.79
S$10899
  Bottom 0: 83.23,41.79 83.55,41.94
S$10900
  Bottom 0: 83.55,41.94 83.82,42.16
S$10901
  Bottom 0: 83.82,42.16 84.02,42.45
S$10902
  Bottom 0: 84.02,42.45 84.15,42.77
S$10903
  Bottom 0: 84.15,42.77 84.2,43.12
S$10904
  Bottom 0: 84.2,43.12 84.15,43.46
S$10905
  Bottom 0: 84.15,43.46 84.05,43.73
S$10906
  Bottom 0: 84.05,43.73 84.47,44.16
S$10907
  Bottom 0: 84.47,44.16 84.51,44.21
S$10908
  Bottom 0: 84.51,44.21 84.55,44.27
S$10909
  Bottom 0: 84.55,44.27 84.58,44.33
S$10910
  Bottom 0: 84.58,44.33 84.59,44.4
S$10911
  Bottom 0: 84.59,44.4 84.6,44.47
S$10912
  Bottom 0: 84.6,44.47 84.6,58.18
S$10913
  Bottom 0: 84.6,58.18 84.59,58.26
S$10914
  Bottom 0: 84.59,58.26 84.58,58.32
S$10915
  Bottom 0: 84.58,58.32 84.55,58.38
S$10916
  Bottom 0: 84.55,58.38 84.51,58.44
S$10917
  Bottom 0: 84.51,58.44 84.47,58.5
S$10918
  Bottom 0: 84.47,58.5 75.54,67.43
S$10919
  Bottom 0: 75.54,67.43 75.48,67.47
S$10920
  Bottom 0: 75.48,67.47 75.42,67.51
S$10921
  Bottom 0: 75.42,67.51 75.36,67.54
S$10922
  Bottom 0: 75.36,67.54 75.29,67.56
S$10923
  Bottom 0: 75.29,67.56 75.22,67.56
S$10924
  Bottom 0: 75.22,67.56 64.14,67.56
S$10925
  Bottom 0: 64.14,67.56 64.38,67.8
S$10926
  Bottom 0: 64.38,67.8 64.48,67.76
S$10927
  Bottom 0: 64.48,67.76 64.78,67.74
S$10928
  Bottom 0: 64.78,67.74 65.08,67.81
S$10929
  Bottom 0: 65.08,67.81 65.34,67.95
S$10930
  Bottom 0: 65.34,67.95 65.54,68.18
S$10931
  Bottom 0: 65.54,68.18 65.68,68.45
S$10932
  Bottom 0: 65.68,68.45 65.72,68.75
S$10933
  Bottom 0: 65.72,68.75 65.68,69.05
S$10934
  Bottom 0: 65.68,69.05 65.54,69.32
S$10935
  Bottom 0: 65.54,69.32 65.34,69.54
S$10936
  Bottom 0: 65.34,69.54 65.08,69.69
S$10937
  Bottom 0: 65.08,69.69 64.78,69.76
S$10938
  Bottom 0: 64.78,69.76 64.48,69.74
S$10939
  Bottom 0: 64.48,69.74 64.2,69.63
S$10940
  Bottom 0: 64.2,69.63 63.96,69.44
S$10941
  Bottom 0: 63.96,69.44 63.79,69.19
S$10942
  Bottom 0: 63.79,69.19 63.7,68.9
S$10943
  Bottom 0: 63.7,68.9 63.7,68.59
S$10944
  Bottom 0: 63.7,68.59 63.76,68.42
S$10945
  Bottom 0: 63.76,68.42 63.66,68.33
S$10946
  Bottom 0: 63.66,68.33 59.89,68.33
S$10947
  Bottom 0: 59.89,68.33 67.41,75.84
S$10948
  Bottom 0: 67.41,75.84 67.34,75.58
S$10949
  Bottom 0: 67.34,75.58 67.34,75.26
S$10950
  Bottom 0: 67.34,75.26 67.42,74.94
S$10951
  Bottom 0: 67.42,74.94 67.6,74.67
S$10952
  Bottom 0: 67.6,74.67 67.83,74.44
S$10953
  Bottom 0: 67.83,74.44 68.12,74.3
S$10954
  Bottom 0: 68.12,74.3 68.44,74.23
S$10955
  Bottom 0: 68.44,74.23 68.77,74.25
S$10956
  Bottom 0: 68.77,74.25 69.07,74.36
S$10957
  Bottom 0: 69.07,74.36 69.33,74.55
S$10958
  Bottom 0: 69.33,74.55 69.54,74.8
S$10959
  Bottom 0: 69.54,74.8 69.67,75.1
S$10960
  Bottom 0: 69.67,75.1 69.69,75.22
S$10961
  Bottom 0: 69.69,75.22 74.09,75.22
S$10962
  Bottom 0: 74.09,75.22 74,74.98
S$10963
  Bottom 0: 74,74.98 74,74.73
S$10964
  Bottom 0: 74,74.73 74.09,74.5
S$10965
  Bottom 0: 74.09,74.5 74.24,74.34
S$10966
  Bottom 0: 74.24,74.34 74.24,72.92
S$10967
  Bottom 0: 74.24,72.92 74.24,72.85
S$10968
  Bottom 0: 74.24,72.85 74.26,72.78
S$10969
  Bottom 0: 74.26,72.78 74.28,72.72
S$10970
  Bottom 0: 74.28,72.72 74.32,72.66
S$10971
  Bottom 0: 74.32,72.66 74.36,72.61
S$10972
  Bottom 0: 74.36,72.61 84.99,61.98
S$10973
  Bottom 0: 84.99,61.98 84.99,41.23
S$10974
  Bottom 0: 84.99,41.23 76.88,33.12
S$10975
  Bottom 0: 76.88,33.12 76.84,33.07
S$10976
  Bottom 0: 76.84,33.07 76.8,33.01
S$10977
  Bottom 0: 76.8,33.01 76.77,32.95
S$10978
  Bottom 0: 76.77,32.95 76.76,32.88
S$10979
  Bottom 0: 76.76,32.88 76.75,32.81
S$10980
  Bottom 0: 76.75,32.81 76.75,26.42
S$10981
  Bottom 0: 76.75,26.42 76.74,26.45
S$10982
  Bottom 0: 76.74,26.45 76.69,26.52
S$10983
  Bottom 0: 76.69,26.52 76.63,26.59
S$10984
  Bottom 0: 76.63,26.59 71.84,31.39
S$10985
  Bottom 0: 71.84,31.39 71.88,31.69
S$10986
  Bottom 0: 71.88,31.69 71.83,32.01
S$10987
  Bottom 0: 71.83,32.01 71.7,32.31
S$10988
  Bottom 0: 71.7,32.31 71.48,32.55
S$10989
  Bottom 0: 71.48,32.55 71.21,32.73
S$10990
  Bottom 0: 71.21,32.73 70.9,32.82
S$10991
  Bottom 0: 70.9,32.82 70.57,32.82
S$10992
  Bottom 0: 70.57,32.82 70.26,32.73
S$10993
  Bottom 0: 70.26,32.73 69.99,32.55
S$10994
  Bottom 0: 69.99,32.55 69.9,32.44
S$10995
  Bottom 0: 69.9,32.44 69.9,33.03
S$10996
  Bottom 0: 69.9,33.03 69.89,33.1
S$10997
  Bottom 0: 69.89,33.1 69.88,33.16
S$10998
  Bottom 0: 69.88,33.16 69.85,33.23
S$10999
  Bottom 0: 69.85,33.23 69.81,33.29
S$11000
  Bottom 0: 69.81,33.29 69.77,33.34
S$11001
  Bottom 0: 69.77,33.34 66.29,36.83
S$11002
  Bottom 0: 66.29,36.83 66.23,36.87
S$11003
  Bottom 0: 66.23,36.87 66.17,36.91
S$11004
  Bottom 0: 66.17,36.91 66.11,36.93
S$11005
  Bottom 0: 66.11,36.93 66.04,36.95
S$11006
  Bottom 0: 66.04,36.95 65.97,36.95
S$11007
  Bottom 0: 65.97,36.95 51.49,36.95
S$11008
  Bottom 0: 51.49,36.95 45.95,42.49
S$11009
  Bottom 0: 45.95,42.49 46.05,42.77
S$11010
  Bottom 0: 46.05,42.77 46.1,43.12
S$11011
  Bottom 0: 46.1,43.12 46.05,43.46
S$11012
  Bottom 0: 46.05,43.46 45.92,43.79
S$11013
  Bottom 0: 45.92,43.79 45.72,44.07
S$11014
  Bottom 0: 45.72,44.07 45.45,44.3
S$11015
  Bottom 0: 45.45,44.3 45.13,44.45
S$11016
  Bottom 0: 45.13,44.45 44.79,44.51
S$11017
  Bottom 0: 44.79,44.51 44.44,44.49
S$11018
  Bottom 0: 44.44,44.49 44.1,44.38
S$11019
  Bottom 0: 44.1,44.38 43.81,44.19
S$11020
  Bottom 0: 43.81,44.19 43.57,43.94
S$11021
  Bottom 0: 43.57,43.94 43.4,43.63
S$11022
  Bottom 0: 43.4,43.63 43.31,43.29
S$11023
  Bottom 0: 43.31,43.29 43.31,42.94
S$11024
  Bottom 0: 43.31,42.94 43.4,42.6
S$11025
  Bottom 0: 43.4,42.6 43.57,42.29
S$11026
  Bottom 0: 43.57,42.29 43.81,42.04
S$11027
  Bottom 0: 43.81,42.04 44.1,41.85
S$11028
  Bottom 0: 44.1,41.85 44.44,41.74
S$11029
